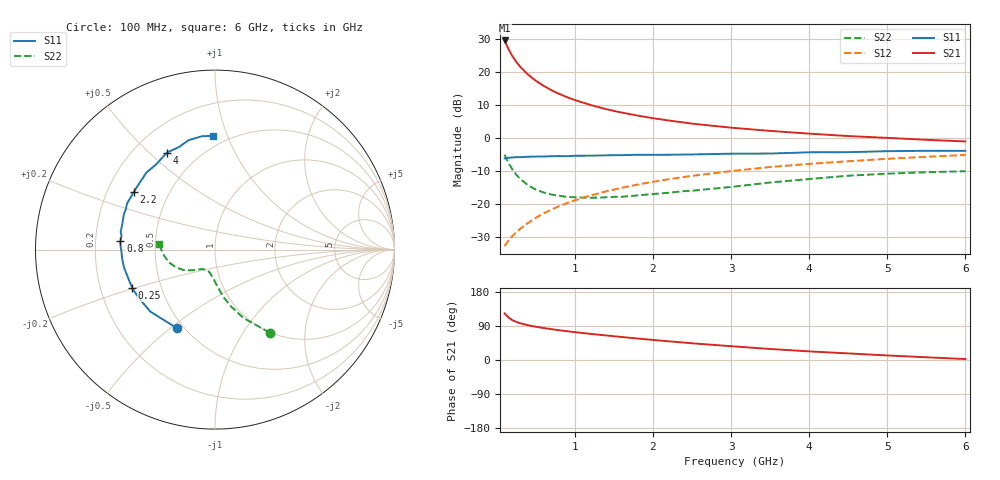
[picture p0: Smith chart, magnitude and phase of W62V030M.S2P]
! SIEMENS Small Signal Semiconductors
! BFR193W
! Si NPN RF Bipolar Junction Transistor in SOT323
! VCE = 2 V  IC = 30 mA
! Common Emitter S-Parameters:  September  1992
# GHz  S  MA  R  50
!  f  S11  S21  S12  S22
! GHz  MAG  ANG  MAG  ANG  MAG  ANG  MAG  ANG
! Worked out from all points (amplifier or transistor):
!   28 points, 100 MHz to 6 GHz, reference 50 ohm
!   highest |S21| = 29.6 dB at 100 MHz (marker M1)
!   |S21| within 3 dB of that: start of sweep to 158.2 MHz
!   unconditionally stable (mu >= 1): 591.9 MHz to 2.537 GHz
!   at 300 MHz: K = 0.86, MSG = 24.6 dB, |S12| = -27.6 dB
!   at 1.5 GHz: K = 1.04, MAG = 10.8 dB, |S12| = -15.7 dB
!   at 6 GHz: K = 0.92, MSG = 2.0 dB, |S12| = -5.2 dB
!   lowest NFmin = 1.90 dB at 450 MHz
!   S11 on the Smith chart (normalised r, x): 100 MHz: 0.46, -0.53; 250 MHz: 0.34, -0.20; 800 MHz: 0.31, +0.04; 2.2 GHz: 0.31, +0.29; 4 GHz: 0.33, +0.57; 6 GHz: 0.42, +0.89
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0.1  0.4863 -115.9  30.03 123.1  0.0227 58.0  0.5544 -56.6
0.15  0.499 -136.1  22.12 112.1  0.0278 57.5  0.4141 -67.3
0.2  0.503 -147.4  17.34 105.2  0.0324 58.6  0.3309 -74.1
0.25  0.5084 -155.0  14.16 100.6  0.037 60.6  0.2743 -79.3
0.3  0.5086 -160.3  11.97 97.0  0.0417 62.6  0.2389 -82.5
0.4  0.5165 -168.7  9.088 91.7  0.0511 65.5  0.1908 -88.2
0.5  0.5193 -173.8  7.329 87.7  0.0613 67.6  0.1634 -92.6
0.6  0.5211 -178.2  6.144 84.4  0.0715 68.6  0.148 -97.1
0.7  0.5257 178.3  5.267 81.3  0.0816 69.5  0.1378 -100.1
0.8  0.5293 174.8  4.638 78.5  0.092 69.7  0.1323 -103.4
0.9  0.5261 171.9  4.133 76.0  0.1025 69.9  0.1267 -105.9
1  0.5348 169.4  3.747 73.4  0.1128 70.0  0.1252 -108.3
1.2  0.5362 164.2  3.151 69.0  0.1335 69.3  0.1231 -113.9
1.4  0.5421 160.2  2.726 64.8  0.154 68.4  0.1251 -118.0
1.6  0.5455 155.9  2.419 60.7  0.1746 67.4  0.1276 -121.9
2.2  0.5542 144.7  1.833 49.4  0.2353 63.3  0.1466 -130.3
2.5  0.5595 139.5  1.642 44.1  0.2648 61.0  0.1575 -133.9
3.5  0.5774 124.4  1.274 29.1  0.3602 52.4  0.21 -147.4
4  0.6032 116.4  1.158 22.7  0.4026 47.9  0.2369 -154.9
4.5  0.6058 109.3  1.064 17.4  0.4413 43.5  0.266 -164.3
5.5  0.6357 96.7  0.933 7.2  0.5154 34.9  0.3007 179.4
6  0.6344 90.8  0.881 2.5  0.5497 30.4  0.3111 174.6
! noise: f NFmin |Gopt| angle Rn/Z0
0.45  1.9  0.4  180  0.09
0.9  1.95  0.43  -173  0.11
1.8  2.4  0.58  -144  0.24
